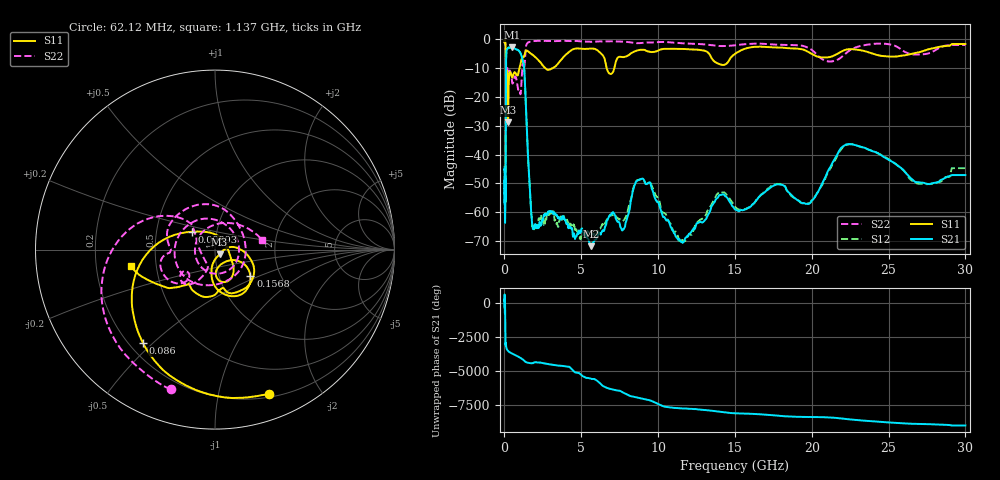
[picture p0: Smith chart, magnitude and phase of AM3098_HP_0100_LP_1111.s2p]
! Date/Time: Thu, Feb 28, 2019 8:35 AM
! Network Analyzer: Agilent Technologies E8364B Rev: A.07.50.67
! Sweep from 0.010 to 30.000 GHz, 1601 Points, Sweep Type: LOG
! Power Supply: 5.022 V, 0.002 A
# Hz S DB R 50
!freq MagS11 AngS11 MagS21 AngS21 MagS12 AngS12 MagS22 AngS22
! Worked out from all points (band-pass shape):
!   1601 points, 10 MHz to 30 GHz, reference 50 ohm
!   highest |S21| = -2.75 dB at 498 MHz (marker M1); lowest = -71.8 dB at 5.64 GHz (marker M2)
!   |S21| within 3 dB of the highest: 112.7 MHz to 1.113 GHz (1 GHz wide, 163 % of centre)
!   lowest |S11| = -28.8 dB at 233.9 MHz (marker M3), VSWR 1.08, Z = 52.5 - j2.74 ohm
!   |S11| at or under -10 dB: 95.98 MHz to 973.3 MHz (877.3 MHz wide, 164 % of centre); 2.668 GHz to 3.133 GHz (465 MHz wide, 16 % of centre); 6.654 GHz to 7.149 GHz (495.3 MHz wide, 7.18 % of centre)
!   |S22| runs from -22.2 to -0.5 dB; largest |S21 - S12| = 0.011
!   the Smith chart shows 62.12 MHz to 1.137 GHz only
!   S11 on the Smith chart (normalised r, x): 62.12 MHz: 0.23, -1.42; 86 MHz: 0.25, -0.46; 98.93 MHz: 0.76, +0.16; 156.8 MHz: 1.41, -0.44; 1.137 GHz: 0.36, -0.09
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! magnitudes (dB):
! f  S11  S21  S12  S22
! 10 MHz  -0.4  -45.4  -43.8  -0.6
! 38.04 MHz  -0.5  -61.6  -58.6  -1.0
! 62.12 MHz  -1.3  -50.8  -52.0  -1.8
! 76.26 MHz  -2.1  -52.7  -56.1  -2.5
! 86 MHz  -3.7  -38.2  -38.5  -4.0
! 98.93 MHz  -15.8  -12.9  -12.9  -19.9
! 144.7 MHz  -16.6  -3.7  -3.6  -13.5
! 156.8 MHz  -12.2  -3.5  -3.5  -11.4
! 233.9 MHz  -28.8  -2.9  -2.9  -11.9
! 498 MHz  -13.2  -2.8  -2.7  -15.0
! 550.5 MHz  -12.7  -2.9  -2.9  -15.1
! 1.137 GHz  -6.4  -6.2  -6.2  -11.4
! 1.308 GHz  -5.4  -12.2  -12.1  -8.9
! 1.793 GHz  -5.2  -63.7  -63.5  -0.6
! 2.084 GHz  -6.5  -65.1  -65.0  -0.5
! 5.64 GHz  -3.2  -71.8  -67.8  -0.8
! 7.926 GHz  -5.9  -63.1  -61.2  -0.8
! 9.118 GHz  -3.6  -49.3  -49.3  -1.1
! 11.77 GHz  -3.3  -68.9  -70.0  -1.4
! 19.7 GHz  -4.2  -57.1  -57.0  -2.7
! 22.56 GHz  -3.4  -36.4  -36.4  -3.5
! 30 GHz  -1.6  -47.1  -44.7  -1.9
